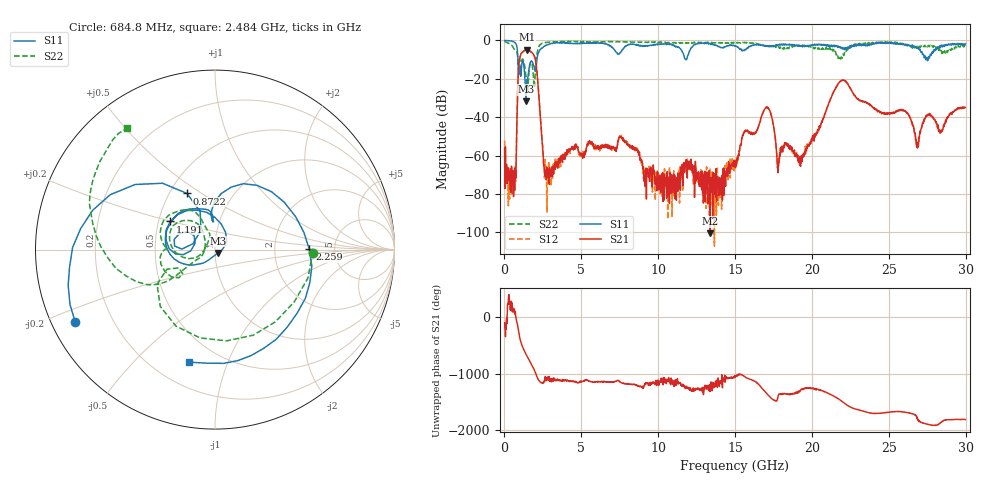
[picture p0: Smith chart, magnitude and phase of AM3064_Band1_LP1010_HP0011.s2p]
# Hz S DB R 50.0
!freq dBS11 angS11 dBS21 angS21 dBS12 angS12 dBS22 angS22
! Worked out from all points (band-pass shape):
!   1600 points, 10 MHz to 29.98 GHz, reference 50 ohm
!   highest |S21| = -4.80 dB at 1.453 GHz (marker M1); lowest = -100.5 dB at 13.37 GHz (marker M2)
!   |S21| within 3 dB of the highest: 1.039 GHz to 1.923 GHz (883.6 MHz wide, 59.7 % of centre)
!   lowest |S11| = -31.7 dB at 1.397 GHz (marker M3), VSWR 1.05, Z = 51.9 - j1.89 ohm
!   |S11| at or under -10 dB: 876.6 MHz to 2.11 GHz (1.233 GHz wide, 82.6 % of centre); 11.79706 GHz to 11.83926 GHz (42.2 MHz wide, 0.357 % of centre); 27.41292 GHz to 27.43522 GHz (22.29 MHz wide, 0.0813 % of centre)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
!   |S22| runs from -25.7 to -0.4 dB; largest |S21 - S12| = 0.0077
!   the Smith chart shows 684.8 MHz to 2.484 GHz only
!   S11 on the Smith chart (normalised r, x): 684.8 MHz: 0.07, -0.24; 872.2 MHz: 0.61, +0.44; 1.191 GHz: 0.58, +0.20; 2.259 GHz: 3.21, +0.01; 2.484 GHz: 0.34, -0.74
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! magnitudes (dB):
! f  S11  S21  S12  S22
! 10 MHz  0.0  -55.8  -52.2  -0.4
! 328.6 MHz  -0.2  -73.4  -82.8  -1.7
! 684.8 MHz  -1.1  -66.5  -68.2  -5.3
! 872.2 MHz  -9.1  -22.7  -22.7  -10.8
! 1.191 GHz  -10.6  -6.1  -6.0  -9.7
! 1.397 GHz  -31.7  -4.8  -4.8  -18.8
! 1.453 GHz  -22.1  -4.8  -4.7  -21.5
! 2.259 GHz  -5.6  -31.3  -31.2  -2.8
! 2.484 GHz  -3.8  -56.5  -54.7  -1.6
! 2.878 GHz  -2.1  -68.8  -63.1  -0.9
! 5.015 GHz  -1.4  -59.8  -60.1  -0.7
! 7.582 GHz  -6.0  -50.7  -49.5  -0.5
! 10 GHz  -2.0  -71.3  -71.2  -1.0
! 13.37 GHz  -1.6  -100.5  -67.0  -1.1
! 15 GHz  -2.9  -62.8  -63.7  -1.5
! 17.05 GHz  -2.8  -34.7  -34.8  -3.3
! 17.82 GHz  -2.2  -65.0  -63.8  -3.3
! 19.99 GHz  -2.8  -52.4  -52.9  -3.3
! 21.94 GHz  -4.1  -20.9  -20.9  -9.4
! 25 GHz  -1.1  -38.0  -38.1  -1.0
! 26.87 GHz  -4.1  -55.3  -55.4  -3.2
! 29.98 GHz  -1.8  -34.9  -35.2  -3.1
